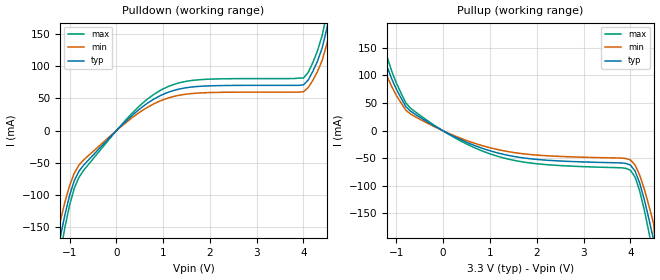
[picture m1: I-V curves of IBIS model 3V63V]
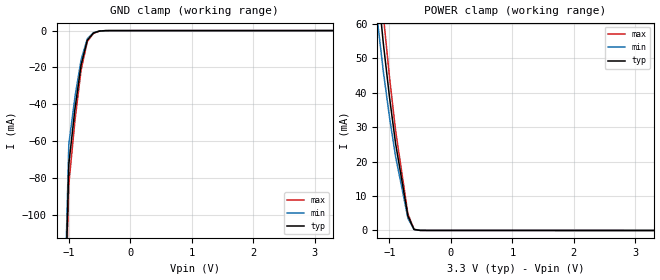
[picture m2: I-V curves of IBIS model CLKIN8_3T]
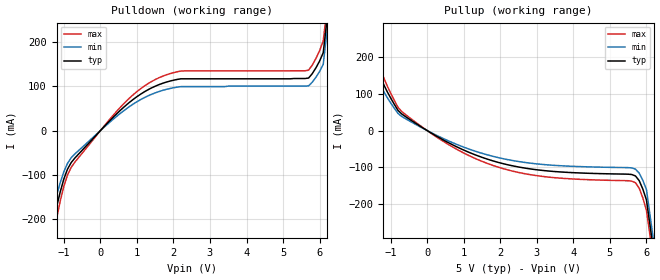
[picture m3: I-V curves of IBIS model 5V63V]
[IBIS Ver]   2.1
[File name]   512_3_5.ibs
[File Rev]   2.0
[Date]   06/5/2000
[Source]   ICS MicroClock Applications Engineering 2
[Disclaimer] This information is for modeling purposes only, and is
(C) Copyright Integrated Circuit Systems, Inc. 1997-2001
   All rights reserved
ICS hereby grants the user of this IBIS model a non-exclusive,
nontransferable license to use this IBIS model under the following terms.
Before using this IBIS model, the user should read this license.
If the user does not accept these terms,  the IBIS model should be
returned to ICS within 30 days.
   The user is granted this license only to use the IBIS model and
is not granted rights to sell, load, rent, lease or license the IBIS
model in whole or in part, or in modified form to anyone other than
user. User may modify the IBIS model to suit its specific
applications but rights to derivative works and such modifications
shall belong to ICS.
   This IBIS model is provided on an "AS IS" basis and ICS makes
absolutely no warranty with respect to the information contained
herein. ICS DISCLAIMS AND CUSTOMER WAIVES ALL WARRANTIES, EXPRESS
OR IMPLIED, INCLUDING WARRANTIES OF MERCHANTABILITY OR FITNESS FOR
A PARTICULAR PURPOSE. The entire risk as to quality and performance
is with the Customer. ACCORDINGLY, IN NO EVENT SHALL THE COMPANY BE
LIABLE FOR ANY DAMAGES, WHETHER IN CONTRACT OR TORT,INCLUDING ANY
LOST PROFITS OR OTHER INCIDENTAL, CONSEQUENTIAL, EXEMPLARY, OR
PUNITIVE DAMAGES ARISING OUT OF THE USE OR APPLICATION OF THE IBIS
model provided in this package. Further, ICS reserves the right to
make changes without notice to any product herein to improve
reliability, function, or design. ICS does not convey any license
under patent rights or any other intellectual property rights,
including those of third parties.
   ICS is not obligated to provide maintenance or support
for the licensed IBIS model.
[Component]   ICS512_3v
[Manufacturer] Integrated Circuit Systems Inc.
[Package]
|   typ   min   max
R_pkg   40m   35m   45m
L_pkg   1.65nH   1.35nH   1.95nH
C_pkg   0.24pF   0.14pF   0.34pF
[pin]   signal_name   model_name   R_pin   L_pin   C_pin
   1   X1/ICLK   CLKIN8_3T
   2   VDD   nc
   3   GND   nc
   4   REF   3V63V
   5   CLK   3V63V
   6   S0   CLKIN8_3T
   7   S1   CLKIN8_3T
   8   X2   nc
[Component]   ICS512_5v
[Manufacturer] Integrated Circuit Systems Inc.
[Package]
|   typ   min   max
R_pkg   40m   35m   45m
L_pkg   1.65nH   1.35nH   1.95nH
C_pkg   0.24pF   0.14pF   0.34pF
[pin]   signal_name   model_name   R_pin   L_pin   C_pin
   1   X1/ICLK   CLKIN8_3T
   2   VDD   nc
   3   GND   nc
   4   REF   5V63V
   5   CLK   5V63V
   6   S0   CLKIN8_5T
   7   S1   CLKIN8_5T
   8   X2   nc
| Models and submodels in the file (4): 3V63V (Output), CLKIN8_3T (Input), 5V63V (Output), CLKIN8_5T (Input)
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|   ICS512 3.3V Clock Drive Model
| This model is suitable for all output pins on the
| ICS512
[Model]   3V63V
Model_type   Output
Polarity   Non-Inverting
Vmeas =   1.40V
|   typ   min   max
C_comp   5pF   4pF   6pF
|   typ   min   max
[Voltage range]  3.3V   3.15V   3.45V
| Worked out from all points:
|   slope of the pulldown table from 0 to 0.495 V, typ, clamps not added: 14.9 ohm
|   slope of the pullup table from 0 to 0.495 V, typ, clamps not added: 24.2 ohm
[pulldown]
|Voltage I (typ)   I (min)   I (max)
-3.3V     -3A        -3A        -3A
-1.3V     -199.9mA   -169.9mA   -229.9mA
-1.2V     -166.1mA   -141.2mA   -191mA
-1.1V     -131mA     -111.3mA   -150.6mA
-800mV    -63.14mA   -53.66mA   -72.61mA
400mV     27.29mA    23.2mA     31.39mA
1.1V      58.96mA    50.11mA    67.8mA
4V        70.65mA    60.05mA    81.25mA
4.3V      107.5mA    91.34mA    123.6mA
4.5V      157.8mA    134.1mA    181.5mA
4.6V      195.8mA    166.4mA    225.2mA
6.6V      3A         3A         3A
[pullup]
|Voltage I (typ)   I (min)   I (max)
-3.3V     3A         3A         3A
-1.4V     190.5mA    161.9mA    219.1mA
-1.3V     149.2mA    126.8mA    171.6mA
-1.2V     116.4mA    98.91mA    133.8mA
-800mV    43.62mA    37.08mA    50.17mA
400mV     -17.51mA   -14.88mA   -20.14mA
1.6V      -48.26mA   -41.02mA   -55.49mA
4V        -62.64mA   -53.25mA   -72.04mA
4.2V      -95.46mA   -81.14mA   -109.8mA
4.4V      -161.7mA   -137.4mA   -185.9mA
4.5V      -199.9mA   -169.9mA   -229.9mA
6.6V      -3A        -3A        -3A
[Ramp]
|   typ   min   max
dV/dt_r   1.31/0.41n   1.14/0.45n   1.37/0.37n
dV/dt_f   1.54/0.34n   1.42/0.38n   1.62/0.31n
|   0.6 um mask 3.3V  INPUT  Model
| This model is suitable for CLK INPUT Pin ( TTL level)  on the
| 0.8 um mask set product
[Model]   CLKIN8_3T
Model_type   Input
|   typ   min   max
C_comp   5pF   4pF   6pF
Vinl =0.8V   | Input logic  "low" DC voltage
Vinh=2.0V   | Input logic  "high" DC voltage
|   typ   min   max
[Voltage range]  3.3V   3.15V   3.45V
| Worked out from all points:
|   GND clamp passes 1 mA (typ) near -0.57 V on its own axis
|   POWER clamp passes 1 mA (typ) near -0.62 V on its own axis
[GND_clamp]
|Voltage I (typ)   I (min)   I (max)
-3.3V     -3A        -3A        -3A
-1V       -72.57mA   -61.68mA   -83.45mA
-900mV    -42.4mA    -36.04mA   -48.76mA
-800mV    -18.58mA   -15.79mA   -21.37mA
-700mV    -5.28mA    -4.49mA    -6.07mA
-600mV    -1.34mA    -1.14mA    -1.54mA
-500mV    -240uA     -200uA     -270uA
-400mV    -20.8uA    -18uA      -24uA
3.3V      6.8uA      5.78uA     7.82uA
[POWER_clamp]
|Voltage I (typ)   I (min)   I (max)
-3.3V     3A         3A         3A
-1.2V     72.62mA    61.73mA    83.52mA
-1.1V     54.43mA    46.27mA    62.6mA
-1V       38.85mA    33.02mA    44.68mA
-900mV    25.25mA    21.46mA    29.03mA
-700mV    4.221mA    3.588mA    4.854mA
-600mV    294uA      250uA      338uA
-400mV    10.3uA     8.73uA     11.8uA
3.3V      -6.44uA    -5.5uA     -7.4uA
|   ICS512 5V Clock Drive Model
| This model is suitable for all output pins on the
| ICS512
[Model]   5V63V
Model_type   Output
Polarity   Non-Inverting
Vmeas =   2.30V
|   typ   min   max
C_comp   5pF   4pF   6pF
|   typ   min   max
[Voltage range]  5.0V   4.5V   5.5V
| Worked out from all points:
|   slope of the pulldown table from 0 to 0.75 V, typ, clamps not added: 12.3 ohm
|   slope of the pullup table from 0 to 0.75 V, typ, clamps not added: 18.2 ohm
[pulldown]
|Voltage I (typ)   I (min)   I (max)
-5V       -3A        -3A        -3A
-1.3V     -199.9mA   -169.9mA   -229.9mA
-1V       -110.1mA   -93.58mA   -126.6mA
-800mV    -72.82mA   -61.89mA   -83.74mA
700mV     57.21mA    48.63mA    65.79mA
1.2V      87.58mA    74.44mA    100.7mA
1.7V      107mA      90.96mA    123.1mA
2.3V      117.3mA    99.6mA     135.3mA
5.7V      119.1mA    101.3mA    137mA
5.9V      142.1mA    120.8mA    163.4mA
6.1V      176.4mA    150mA      202.9mA
10V       3A         3A         3A
[pullup]
|Voltage I (typ)   I (min)   I (max)
-5V       3A         3A         3A
-1.4V     185.7mA    157.9mA    213.6mA
-1.3V     150.3mA    127.8mA    172.9mA
-1.1V     105.9mA    90.04mA    121.8mA
-700mV    44.96mA    38.22mA    51.71mA
500mV     -28.73mA   -24.42mA   -33.04mA
1.6V      -76.04mA   -64.63mA   -87.44mA
3.1V      -107.5mA   -91.34mA   -123.6mA
5.6V      -119.2mA   -101.3mA   -137.1mA
5.8V      -135.5mA   -115.2mA   -155.9mA
6V        -188mA     -159.8mA   -216.2mA
10V       -3A        -3A        -3A
[Ramp]
|   typ   min   max
dV/dt_r   2.21/0.40n   1.90/0.44n   2.32/0.36n
dV/dt_f   2.48/0.36n   2.16/0.39n   2.60/0.32n
